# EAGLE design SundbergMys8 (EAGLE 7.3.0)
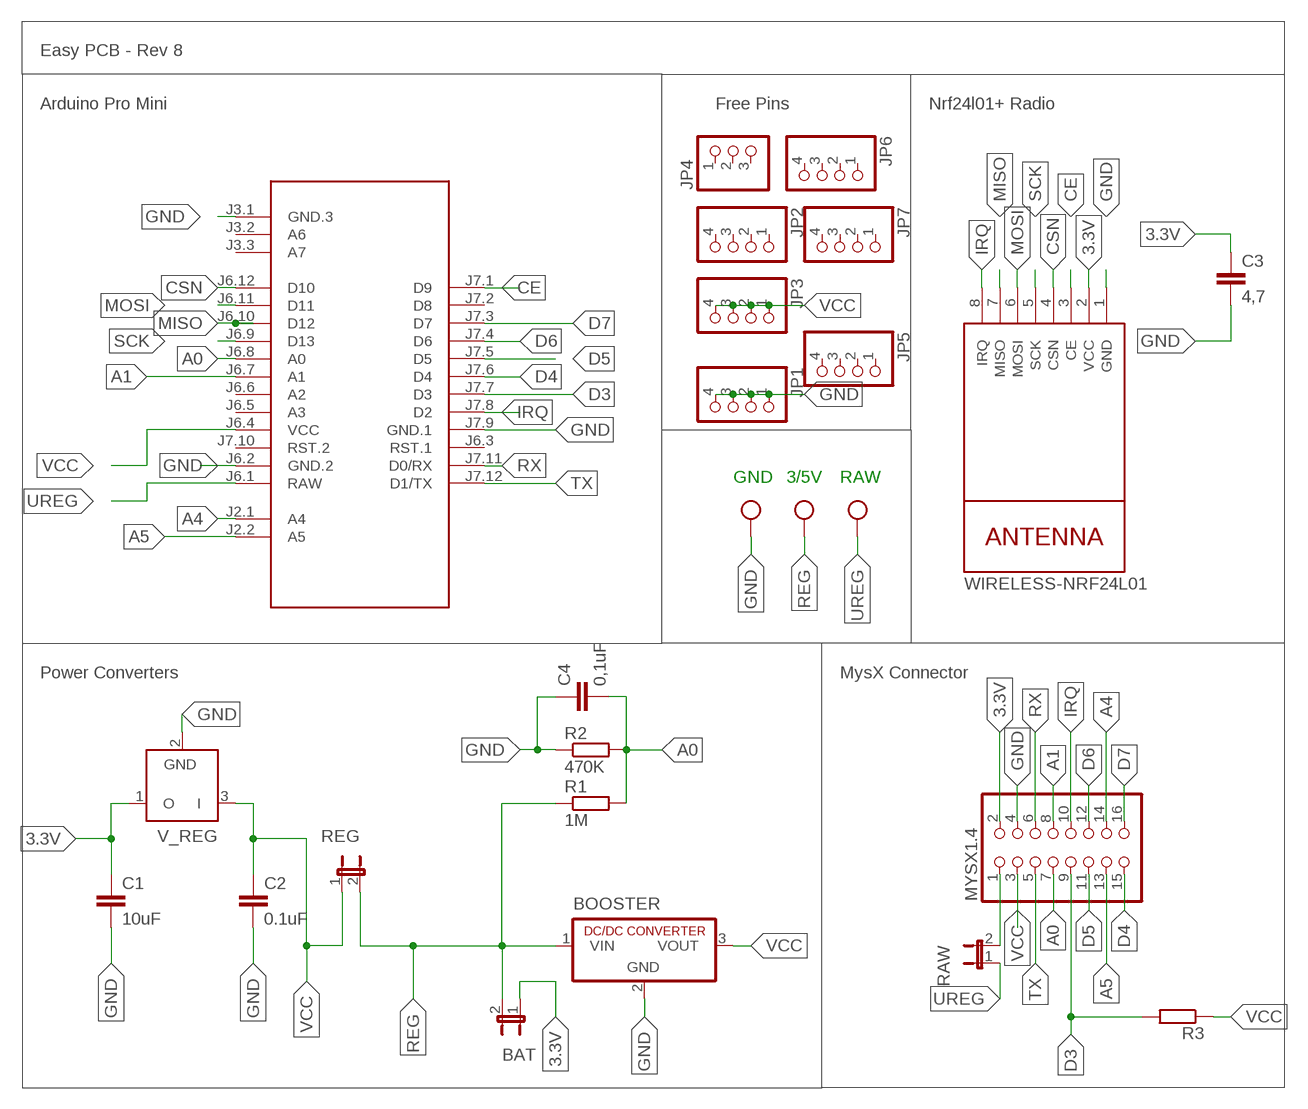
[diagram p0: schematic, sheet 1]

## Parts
.  W237-103  [W237-103]
BAT  JP1E  [JP1]
BOOSTER  R-78C1.8-1.0  [SIP3]
C1  10uF  C5/2.5  [C5B2.5]
C2  0.1uF  C5/2.5  [C5B2.5]
C3  4,7  C5/2.5  [C5B2.5]
C4  0,1uF  C5/2.5  [C5B2.5]
JP1  PINHD-1X04_2.54-S  [1X04-S]
JP2  PINHD-1X04_2.54-S  [1X04-S]
JP3  PINHD-1X04_2.54-S  [1X04-S]
JP4  PINHD-1X03_2.54-S  [1X03-S]
JP5  PINHD-1X04_2.54-S  [1X04-S]
JP6  PINHD-1X04_2.54-S  [1X04-S]
JP7  PINHD-1X04_2.54-S  [1X04-S]
M1  ARDUINO-PRO-MINI-3.3V#NP  [ARDUINO-PRO-MINI#NP]
MYSX1.4  PINHD-2X08_2.54  [2X08]
NRF24L01+  WIRELESS-NRF24L01  [WIRELESS-NRF24L01]
R1  1M  R-EU_0204/7  [0204/7]
R2  470K  R-EU_0204/7  [0204/7]
R3  R-EU_0204/7  [0204/7]
RAW  JP1E  [JP1]
REG  JP1E  [JP1]
V_REG  LP2950Z  [TO92]

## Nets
3.3V: BAT.1 C1.1 C3.1 MYSX1.4.2 NRF24L01+.2(VCC) V_REG.1(O)
A0: C4.2 M1.J6.8(A0) MYSX1.4.7 R1.2 R2.2
A1: M1.J6.7(A1) MYSX1.4.8
A4: M1.J2.1(A4) MYSX1.4.14
A5: M1.J2.2(A5) MYSX1.4.13
CE: M1.J7.1(D9) NRF24L01+.3(CE)
CSN: M1.J6.12(D10) NRF24L01+.4(CSN)
D3: M1.J7.7(D3) MYSX1.4.9 R3.2
D4: M1.J7.6(D4) MYSX1.4.15
D5: M1.J7.5(D5) MYSX1.4.11
D6: M1.J7.4(D6) MYSX1.4.12
D7: M1.J7.3(D7) MYSX1.4.16
GND: ..3 BOOSTER.2(GND) C1.2 C2.2 C3.2 C4.1 JP1.1 JP1.2 JP1.3 JP1.4 M1.J3.1(GND.3) M1.J6.2(GND.2) M1.J7.9(GND.1) MYSX1.4.4 NRF24L01+.1(GND) R2.1 V_REG.2(GND)
IRQ: M1.J7.8(D2) MYSX1.4.10 NRF24L01+.8(IRQ)
MISO: M1.J6.10(D12) NRF24L01+.7(MISO)
MOSI: M1.J6.11(D11) NRF24L01+.6(MOSI)
N$1: MYSX1.4.1 RAW.2
REG: ..2 BAT.2 BOOSTER.1(VIN) R1.1 REG.2
RX: M1.J7.11(D0/RX) MYSX1.4.6
SCK: M1.J6.9(D13) NRF24L01+.5(SCK)
TX: M1.J7.12(D1/TX) MYSX1.4.5
UREG: ..1 M1.J6.1(RAW) RAW.1
VCC: BOOSTER.3(VOUT) C2.1 JP3.1 JP3.2 JP3.3 JP3.4 M1.J6.4(VCC) MYSX1.4.3 R3.1 REG.1 V_REG.3(I)
Unconnected: JP2.1 JP2.2 JP2.3 JP2.4 JP4.1 JP4.2 JP4.3 JP5.1 JP5.2 JP5.3 JP5.4 JP6.1 JP6.2 JP6.3 JP6.4 JP7.1 JP7.2 JP7.3 JP7.4 M1.J3.2(A6) M1.J3.3(A7) M1.J6.3(RST.1) M1.J6.5(A3) M1.J6.6(A2) M1.J7.2(D8) M1.J7.10(RST.2)

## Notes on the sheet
- Easy PCB - Rev 8
- Arduino Pro Mini | Free Pins | Nrf24l01+ Radio
- GND | 3/5V | RAW
- Power Converters | MysX Connector

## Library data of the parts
. = con-wago-500:W237-103: WAGO SCREW CLAMP; MPN: 237-103; OC_FARNELL: unknown; OC_NEWARK: 18M7116
BAT RAW REG = jumper:JP1E: JUMPER
BOOSTER = dc-dc-converter:R-78C*-1.0: INNOLINE DC/DC-Converter 1.0 AMP SIP3 Single Output Source: Data sheet
C1-C4 = capacitor-wima:C: CAPACITOR
JP1-JP3 JP5-JP7 = pinhead-2:PINHD-1X04: PIN HEADER
JP4 = pinhead-2:PINHD-1X03: PIN HEADER
M1 = diy-modules:ARDUINO-PRO-MINI-*#NP: Arduino Pro Mini without programming pads
MYSX1.4 = pinhead-2:PINHD-2X08: PIN HEADER
NRF24L01+ = diy-modules:WIRELESS-NRF24L01: 2.4 GHz Wireless Module based on NRF24L01 chip
R1-R3 = rcl:R-EU_: RESISTOR, European symbol
V_REG = linear:LP2950: 100 mA, Low Power Low Dropout Voltage Regulator Source: http://www.onsemi.com/pub/Collateral/LP2950-D.PDF

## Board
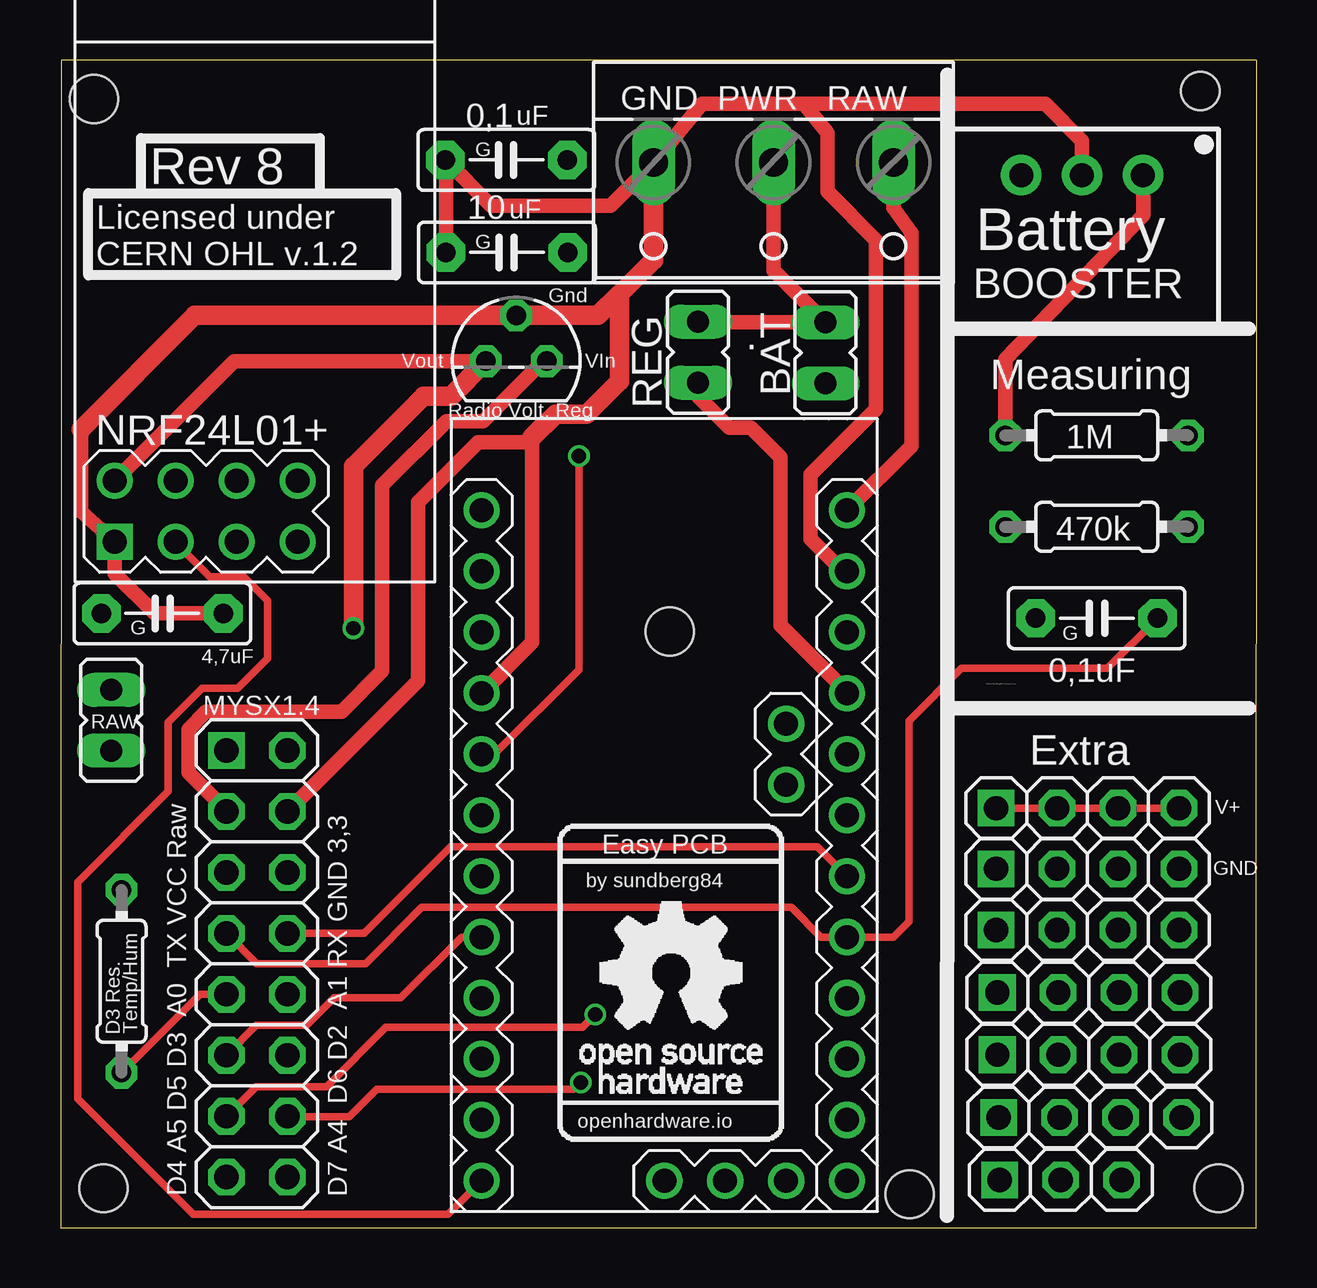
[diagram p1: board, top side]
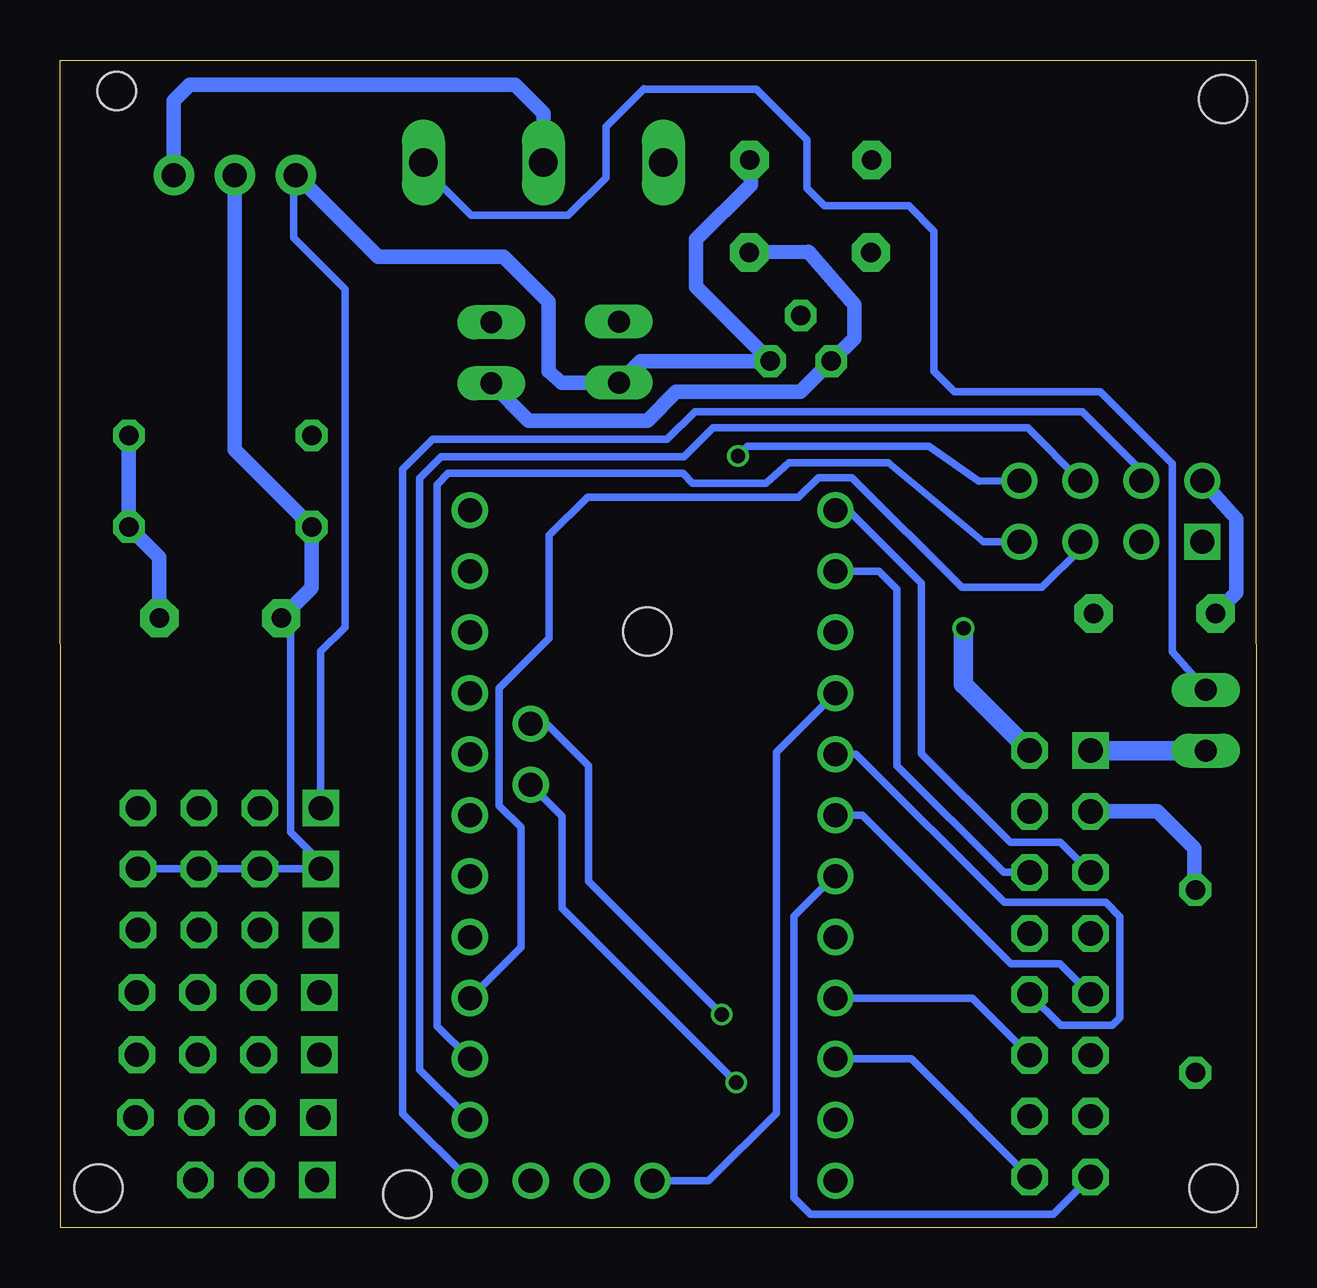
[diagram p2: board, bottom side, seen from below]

Size 49.86 x 48.66 mm. Coordinates in mm from the lower left corner, seen from the top.
Outline: 0,0 49.84,0 49.86,48.66 0.03,48.66 0,0
Copper layers (1*16): Top 0.035mm / dielectric 1.5mm / Bottom 0.035mm
Design rules "dirt_cheap_dirty_boards.v1": minimum track width 5mil, minimum drill 12mil, track to track 5mil, track to pad 5mil, pad to pad 5mil, via to via 5mil, smd to smd 0mil, copper to edge 10mil, drill to drill 10mil, minimum pad ring 10mil, minimum via ring 6mil, stop-mask expansion 2mil, vias tented up to drill 25mil, thermal gap 10mil
Holes 2 mm at 1.78,1.65 48.26,1.65 1.39,47.03 25.39,24.85 35.38,1.4
Holes 1.6 mm at 47.5,47.37

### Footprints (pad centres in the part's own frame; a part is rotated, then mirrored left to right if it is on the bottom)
W237-103 = drill 1.194 long: 1 -5,-1.29; 2 0,-1.29; 3 5,-1.29
JP1 = drill 0.914 long: 1 0,-1.27; 2 0,1.27
SIP3 = drill 1 pad 1.676: 1 -2.54,0; 2 0,0; 3 2.54,0
C5B2.5 = drill 0.813 pad 1.6 octagon: 1 -2.54,0; 2 2.54,0
1X04-S = drill 1.016 square: 1 -3.81,0 | drill 1.016 octagon: 2 -1.27,0; 3 1.27,0; 4 3.81,0
1X03-S = drill 1.016 square: 1 -2.54,0 | drill 1.016 octagon: 2 0,0; 3 2.54,0
ARDUINO-PRO-MINI#NP = drill 1: J2.1 -1.27,5.08; J2.2 -3.81,5.08; J3.1 15.24,0; J3.2 15.24,2.54; J3.3 15.24,5.08; J6.1 -12.7,7.62; J6.2 -10.16,7.62; J6.3 -7.62,7.62; J6.4 -5.08,7.62; J6.5 -2.54,7.62; J6.6 0,7.62; J6.7 2.54,7.62; J6.8 5.08,7.62; J6.9 7.62,7.62; J6.10 10.16,7.62; J6.11 12.7,7.62; J6.12 15.24,7.62; J7.1 15.24,-7.62; J7.2 12.7,-7.62; J7.3 10.16,-7.62; J7.4 7.62,-7.62; J7.5 5.08,-7.62; J7.6 2.54,-7.62; J7.7 0,-7.62; J7.8 -2.54,-7.62; J7.9 -5.08,-7.62; J7.10 -7.62,-7.62; J7.11 -10.16,-7.62; J7.12 -12.7,-7.62
2X08 = drill 1.016 square: 1 -8.89,-1.27 | drill 1.016 octagon: 2 -8.89,1.27; 3 -6.35,-1.27; 4 -6.35,1.27; 5 -3.81,-1.27; 6 -3.81,1.27; 7 -1.27,-1.27; 8 -1.27,1.27; 9 1.27,-1.27; 10 1.27,1.27; 11 3.81,-1.27; 12 3.81,1.27; 13 6.35,-1.27; 14 6.35,1.27; 15 8.89,-1.27; 16 8.89,1.27
WIRELESS-NRF24L01 = drill 1 square: 1 -12.7,6.35 | drill 1: 2 -10.16,6.35; 3 -12.7,3.81; 4 -10.16,3.81; 5 -12.7,1.27; 6 -10.16,1.27; 7 -12.7,-1.27; 8 -10.16,-1.27
0204/7 = drill 0.813 octagon: 1 -3.81,0; 2 3.81,0
TO92 = drill 0.813 octagon: 1 -1.27,0; 2 0,1.905; 3 1.27,0

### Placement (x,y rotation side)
.  29.71,43.09 180 top
BAT  31.88,36.46 0 top
BOOSTER  42.57,43.87 180 top
C1  18.6,40.64 180 top
C2  18.57,44.5 180 top
C3  4.24,25.6 0 top
C4  43.18,25.4 0 top
JP1  42.8,14.96 0 top
JP2  42.8,12.41 0 top
JP3  42.8,17.49 0 top
JP4  41.68,2 0 top
JP5  42.85,9.8 0 top
JP6  42.85,7.21 0 top
JP7  42.9,4.6 0 top
M1  25.16,17.2 270 top
MYSX1.4  8.18,11 270 top
NRF24L01+  8.6,41.28 90 top
R1  43.18,33.02 0 top
R2  43.18,29.21 0 top
R3  2.54,10.28 270 top
RAW  2.1,21.15 180 top
REG  26.56,36.48 0 top
V_REG  18.98,36.11 0 top

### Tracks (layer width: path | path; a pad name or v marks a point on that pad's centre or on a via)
3.3V  (via drill 0.6)
  Top 0.61: V_REG.1 7.24,36.11 NRF24L01+.2
  Top 0.813: v12.2,24.99 12.2,31.74 15.12,34.66 16.27,34.66 V_REG.1
  Bottom 0.61: BAT.1 30.32,33.64 25.38,33.64 24.18,34.84 18.99,34.84 V_REG.1 16.75,37.08 16.75,38.46 18.66,40.67 C1.1 | NRF24L01+.2 0.82,29.55 0.82,26.47 C3.1
  Bottom 0.813: MYSX1.4.2 12.2,22.64 v12.2,24.99
A0
  Top 0.305: C4.2 43.63,23.31 37.55,23.31 35.35,21.11 35.35,12.76 34.71,12.12 M1.J6.8 31.69,12.12 30.45,13.36 15.05,13.36 12.7,11.01 8.17,11.01 MYSX1.4.7
  Bottom 0.61: C4.2 45.72,27.94 R2.2 R1.2
A1
  Top 0.305: MYSX1.4.8 12.64,12.27 16.25,15.89 31.55,15.89 M1.J6.7
A4  (via drill 0.6)
  Top 0.305: MYSX1.4.14 9.46,4.64 12.03,4.64 13.18,5.79 21.4,5.79 v21.68,6.06
  Bottom 0.305: v21.68,6.06 28.93,13.31 28.93,17.16 M1.J2.1
A5  (via drill 0.6)
  Top 0.305: MYSX1.4.13 8.14,5.89 11.07,5.89 13.55,8.36 21.75,8.36 v22.27,8.89
  Bottom 0.305: M1.J2.2 29.57,21.01 27.82,19.26 27.82,14.43 v22.27,8.89
CE
  Top 0.305: M1.J7.1 16.14,0.56 5.53,0.56 0.7,5.39 0.7,14.41 4.47,18.18 4.47,21.06 5.9,22.49 7.38,22.49 8.62,23.74 8.62,26.14 7.62,27.14 6.2,27.14 4.79,28.54 NRF24L01+.3
CSN
  Bottom 0.305: M1.J6.12 35.58,4.75 35.58,31.61 34.33,32.86 24.55,32.86 23.4,34.01 7.25,34.01 4.79,31.55 NRF24L01+.4
D3
  Top 0.305: MYSX1.4.9 5.8,9.73 R3.2
  Bottom 0.305: MYSX1.4.9 8.19,11.01 10.22,11.01 16.41,17.2 M1.J7.7
D4
  Bottom 0.305: MYSX1.4.15 8.46,0.56 18.57,0.56 19.27,1.26 19.27,12.99 18.9,13.36 18.65,13.61 17.6,14.66 M1.J7.6
D5
  Top 0.305: MYSX1.4.11 8.15,8.43 10.25,8.43 11.4,9.59 14.18,9.59 16.71,12.12 M1.J7.5
D6
  Bottom 0.305: MYSX1.4.12 11.83,9.58 M1.J7.4
D7
  Bottom 0.305: MYSX1.4.16 14.37,7.04 M1.J7.3
GND
  Top 0.61: 30.98,46.84 31.95,45.64 31.95,43.19 33.98,41.16 33.98,34.11 31.25,31.39 31.25,28.71 32.6,27.36 M1.J6.2 | 30.98,46.84 26.73,46.84 ..3 22.91,42.59 17.95,42.59 C2.2 16.06,44.47 C1.2 | 30.98,46.84 41.04,46.84 42.57,45.31 BOOSTER.2 | M1.J7.9 19.65,24.39 19.65,32.73 | 19.65,32.73 19.65,32.94 | MYSX1.4.4 14.9,22.8 14.9,30.24 17.4,32.73 19.65,32.73 | 0.85,33.29 0.85,29.84 NRF24L01+.1 2.25,27.26 3.91,25.6 C3.2
  Top 0.813: 19.65,32.94 20.62,33.91 21.93,33.91 23.3,35.29 23.3,38.91 | 23.3,38.91 24.71,40.32 ..3 24.68,44.39 | 23.3,38.91 22.41,38.02 V_REG.2 5.58,38.02 0.85,33.29
  Bottom 0.305: C4.1 40.25,25.01 40.25,16.49 38.99,15.23 JP1.1 JP1.2 JP1.3 JP1.4 | M1.J3.1 22.83,1.96 20,4.79 20,19.81 M1.J7.9
  Bottom 0.61: C4.1 39.37,26.67 R2.1 42.57,32.41 BOOSTER.2
IRQ  (via drill 0.6)
  Top 0.305: M1.J7.8 18.13,19.74 18.13,19.79 21.6,23.26 v21.6,32.16
  Bottom 0.305: NRF24L01+.8 11.56,31.1 13.65,32.56 21.2,32.56 v21.6,32.16 | MYSX1.4.10 8.15,8.43 6,8.43 5.67,8.76 5.67,12.96 6.28,13.56 10.5,13.56 16.68,19.74 M1.J7.8
MISO
  Bottom 0.305: M1.J6.10 34.15,8.41 34.15,30.96 33.67,31.43 23.9,31.43 23.5,31.04 20.43,31.04 19.48,31.89 15.32,31.89 11.38,28.59 NRF24L01+.7
MOSI
  Bottom 0.305: NRF24L01+.6 9.52,33.34 22.65,33.34 23.85,32.14 33.98,32.14 34.88,31.24 34.88,6.6 M1.J6.11
N$1
  Bottom 0.813: RAW.2 6.9,19.88 MYSX1.4.1
REG
  Top 0.61: R1.1 39.37,36.2 45.12,42.2 BOOSTER.1 | REG.2 26.59,37.73 BAT.2 29.71,39.9 ..2
  Bottom 0.61: BOOSTER.1 45.11,46.97 44.45,47.62 30.9,47.62 29.71,46.44 ..2
RX
  Bottom 0.305: M1.J7.11 15.72,27.36 14.97,26.61 14.97,19.26 10.53,14.81 MYSX1.4.6
SCK
  Bottom 0.305: M1.J6.9 30.65,11.7 30.65,16.68 31.55,17.59 31.55,22.49 29.48,24.56 29.48,28.86 27.88,30.43 19.07,30.43 18.25,31.26 16.85,31.26 12.28,26.68 8.93,26.68 7.33,28.28 NRF24L01+.5
TX
  Bottom 0.305: MYSX1.4.5 8.16,16.06 10.25,16.06 13.95,19.76 13.95,26.86 16.99,29.9 M1.J7.12
UREG
  Top 0.61: ..1 34.71,42.5 35.45,41.46 35.45,32.57 M1.J6.1
  Bottom 0.305: ..1 34.21,43.67 32.73,42.19 28.68,42.19 27.1,43.76 27.1,45.89 25.52,47.46 25.5,47.44 20.82,47.44 18.73,45.34 18.73,43.31 18,42.59 14.47,42.59 13.43,41.54 13.43,35.69 12.57,34.84 6.5,34.84 3.5,31.84 3.5,23.99 RAW.1
VCC
  Top 0.305: JP3.1 JP3.2 JP3.3 JP3.4
  Top 0.61: REG.1 26.56,34.65 27.88,33.34 28.77,33.34 30,32.11 30,25.11 32.78,22.33 M1.J6.4 | MYSX1.4.3 6.91,17.38 5.33,18.96 5.33,20.79 6.05,21.51 11.7,21.51 13.4,23.21 13.4,30.93 16.07,33.61 17.6,33.61 20.1,36.11 V_REG.3
  Bottom 0.305: JP3.1 38.99,24.02 37.98,25.04 37.98,39.11 40.12,41.26 40.12,43.77 BOOSTER.3
  Bottom 0.61: BOOSTER.3 40.01,43.87 36.6,40.46 31.38,40.46 29.5,38.59 29.5,35.69 28.95,35.21 28.47,35.21 REG.1 25.67,36.11 V_REG.3 23.35,39.2 23.35,41.19 21.07,43.47 C2.1 | MYSX1.4.3 4.12,17.35 2.58,15.81 2.58,14.13 R3.1

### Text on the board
tPlace: uF | uF | Licensed under / CERN OHL v.1.2 | Gnd | Vout | VIn | Easy PCB | by sundberg84 | openhardware.io
tNames: 0,1 | GND PWR RAW | G | Rev 8 | 10 | G | Battery | Measuring | Radio Volt. Reg | 1M | 470k | G | G | 4,7uF | C:/Users/Sundberg/Desktop/open.bmp | 0,1uF | Extra | V+ | GND | D3 Res. | Temp/Hum | D4 A5 D5 D3 A0 TX VCC Raw | D7 A4 D6 D2 A1 RX GND 3,3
